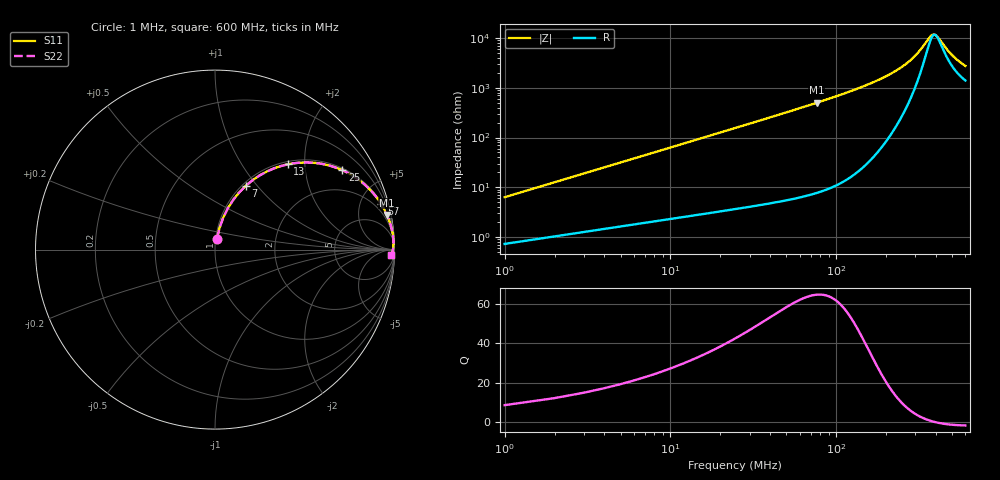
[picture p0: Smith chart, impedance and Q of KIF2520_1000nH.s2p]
!version-2
!date-12.2020
!Series
# MHz S RI R 50
!Freq ReS11 ImS11 ReS21 ImS21 ReS12 ImS12 ReS22 ImS22
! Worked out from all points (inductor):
!   600 points, 1 MHz to 600 MHz, reference 50 ohm
!   read as one part in series: L = 1 uH near 4 MHz
!   highest Q = 64.7 at 76 MHz (marker M1), where L = 1.04 uH
!   self-resonance near 395 MHz
!   S11 on the Smith chart (normalised r, x): 1 MHz: 1.01, +0.13; 7 MHz: 1.04, +0.88; 13 MHz: 1.05, +1.64; 25 MHz: 1.07, +3.15; 57 MHz: 1.12, +7.32; 600 MHz: 29, -47
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1  0.0111 0.0617  0.9889 -0.0617  0.9889 -0.0617  0.0111 0.0617
3  0.0456 0.1777  0.9544 -0.1777  0.9544 -0.1777  0.0456 0.1777
5  0.1019 0.2777  0.8981 -0.2777  0.8981 -0.2777  0.1019 0.2777
7  0.173 0.357  0.827 -0.357  0.827 -0.357  0.173 0.357
10  0.2905 0.436  0.7095 -0.436  0.7095 -0.436  0.2905 0.436
13  0.404 0.4749  0.596 -0.4749  0.596 -0.4749  0.404 0.4749
19  0.5867 0.4792  0.4133 -0.4792  0.4133 -0.4792  0.5867 0.4792
25  0.709 0.4427  0.291 -0.4427  0.291 -0.4427  0.709 0.4427
38  0.8485 0.349  0.1515 -0.349  0.1515 -0.349  0.8485 0.349
57  0.927 0.252  0.073 -0.252  0.073 -0.252  0.927 0.252
76  0.9583 0.1923  0.0417 -0.1923  0.0417 -0.1923  0.9583 0.1923
101  0.9767 0.1431  0.0233 -0.1431  0.0233 -0.1431  0.9767 0.1431
201  0.9938 0.0575  0.00623 -0.0575  0.00623 -0.0575  0.9938 0.0575
259  0.9947 0.0341  0.00532 -0.0341  0.00532 -0.0341  0.9947 0.0341
301  0.9942 0.0214  0.00579 -0.0214  0.00579 -0.0214  0.9942 0.0214
370  0.9923 0.005  0.0077 -0.005  0.0077 -0.005  0.9923 0.005
385  0.9918 0.00196  0.00825 -0.00196  0.00825 -0.00196  0.9918 0.00196
401  0.9911 -0.00114  0.00887 0.00114  0.00887 0.00114  0.9911 -0.00114
460  0.9885 -0.0114  0.0115 0.0114  0.0115 0.0114  0.9885 -0.0114
501  0.9864 -0.0176  0.0136 0.0176  0.0136 0.0176  0.9864 -0.0176
547  0.9839 -0.0238  0.0161 0.0238  0.0161 0.0238  0.9839 -0.0238
600  0.9808 -0.0303  0.0192 0.0303  0.0192 0.0303  0.9808 -0.0303
